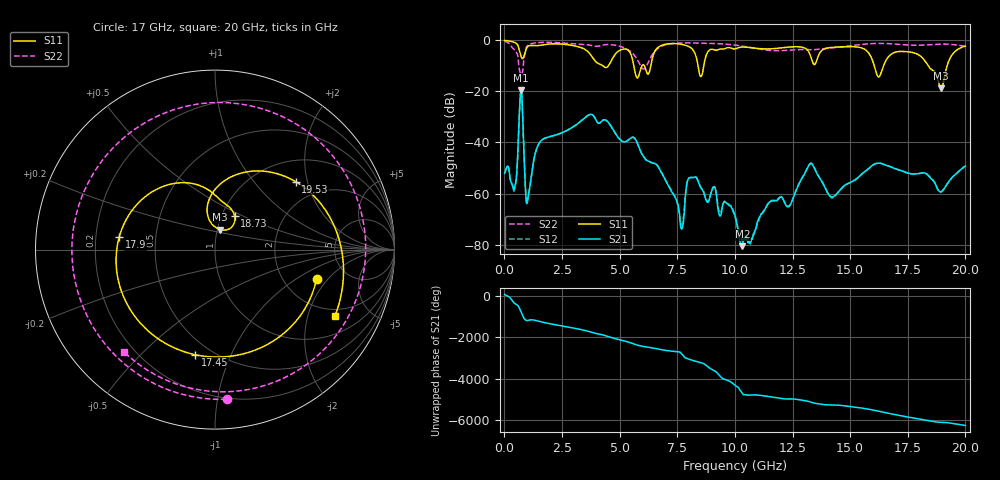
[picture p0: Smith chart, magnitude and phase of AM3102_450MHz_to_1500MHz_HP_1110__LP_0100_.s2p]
!Agilent Technologies,E8364B,MY43040894,A.07.50.67
!Agilent E8364B: A.07.50.67
!Date: Thursday, January 11, 2018 06:43:10
!Correction: S11(Full 2 Port(1,2))
!S21(Full 2 Port(1,2))
!S12(Full 2 Port(1,2))
!S22(Full 2 Port(1,2))
!S2P File: Measurements: S11, S21, S12, S22:
# Hz S  dB  R 50
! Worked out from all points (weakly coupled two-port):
!   1601 points, 10 MHz to 20 GHz, reference 50 ohm
!   highest |S21| = -19.44 dB at 722.1 MHz (marker M1); lowest = -80.6 dB at 10.33 GHz (marker M2)
!   lowest |S11| = -18.8 dB at 18.95 GHz (marker M3), VSWR 1.26, Z = 51.6 + j11.7 ohm
!   |S11| at or under -10 dB: 5.616 GHz to 5.97 GHz (354 MHz wide, 6.11 % of centre); 16.05 GHz to 16.45 GHz (402 MHz wide, 2.47 % of centre); 18.38 GHz to 19.21 GHz (823.7 MHz wide, 4.38 % of centre)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
!   |S22| runs from -13.4 to -0.4 dB; largest |S21 - S12| = 0.0018
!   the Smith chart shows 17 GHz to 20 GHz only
!   S11 on the Smith chart (normalised r, x): 17 GHz: 3.03, -1.52; 17.45 GHz: 0.41, -0.74; 17.9 GHz: 0.30, +0.06; 18.73 GHz: 1.15, +0.45; 19.53 GHz: 1.46, +1.69; 20 GHz: 1.68, -2.99
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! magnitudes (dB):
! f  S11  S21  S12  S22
! 10 MHz  -0.1  -52.0  -52.0  -0.4
! 447.3 MHz  -0.9  -57.3  -57.6  -3.7
! 722.1 MHz  -6.3  -19.4  -19.4  -13.4
! 1.01 GHz  -2.5  -62.2  -62.2  -2.1
! 1.547 GHz  -2.0  -39.8  -39.8  -0.9
! 3.346 GHz  -2.9  -31.4  -31.4  -1.6
! 5.77 GHz  -14.8  -40.3  -40.3  -7.7
! 6.682 GHz  -2.7  -49.6  -49.6  -3.1
! 7.694 GHz  -1.6  -73.9  -72.3  -1.1
! 8.118 GHz  -3.2  -53.7  -53.7  -1.1
! 10.01 GHz  -3.4  -68.7  -69.0  -1.9
! 10.33 GHz  -2.7  -80.6  -78.7  -2.3
! 13.34 GHz  -7.8  -48.3  -48.3  -3.8
! 14.23 GHz  -2.8  -61.2  -61.6  -3.0
! 16.68 GHz  -6.4  -49.3  -49.2  -1.3
! 17 GHz  -4.6  -50.5  -50.3  -1.6
! 17.45 GHz  -4.5  -51.9  -51.8  -1.9
! 17.9 GHz  -5.4  -52.3  -52.3  -2.0
! 18.73 GHz  -13.3  -56.8  -56.9  -1.6
! 18.95 GHz  -18.8  -59.3  -59.4  -1.5
! 19.53 GHz  -4.6  -52.8  -52.8  -1.8
! 20 GHz  -2.3  -49.3  -49.4  -2.3
